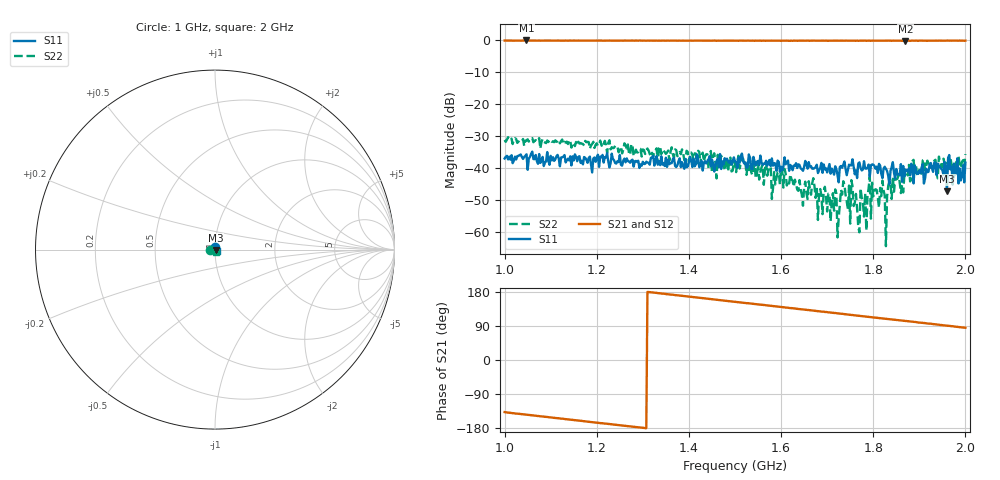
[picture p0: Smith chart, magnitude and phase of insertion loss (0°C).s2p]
!Agilent Technologies,E8363C,MY43030407,A.09.42.15
!Agilent E8363C: A.09.42.15
!Date: Friday, September 05, 2025 17:05:36
!Correction: S11(Full 2 Port(1,2))
!S21(Full 2 Port(1,2))
!S12(Full 2 Port(1,2))
!S22(Full 2 Port(1,2))
!S2P File: Measurements: S11, S21, S12, S22:
# Hz S  dB  R 50
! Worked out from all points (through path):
!   401 points, 1 GHz to 2 GHz, reference 50 ohm
!   highest |S21| = -0.06 dB at 1.048 GHz (marker M1); lowest = -0.2 dB at 1.87 GHz (marker M2)
!   group delay of S21, straight-line fit = 381 ps
!   lowest |S11| = -47.3 dB at 1.96 GHz (marker M3), VSWR 1.01, Z = 50.3 - j0.265 ohm
!   |S11| at or under -10 dB: start of sweep to end of sweep
!   |S22| runs from -64.5 to -30.3 dB; largest |S21 - S12| = 0.011
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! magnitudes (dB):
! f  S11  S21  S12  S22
! 1 GHz  -37.1  -0.1  -0.1  -31.3
! 1.048 GHz  -35.7  -0.1  -0.1  -31.4
! 1.167 GHz  -37.8  -0.1  -0.1  -32.4
! 1.335 GHz  -37.9  -0.1  -0.1  -33.8
! 1.5 GHz  -38.0  -0.1  -0.1  -39.1
! 1.653 GHz  -37.8  -0.1  -0.1  -44.3
! 1.667 GHz  -40.2  -0.1  -0.1  -44.8
! 1.685 GHz  -40.0  -0.1  -0.1  -46.6
! 1.715 GHz  -42.1  -0.1  -0.2  -53.4
! 1.72 GHz  -40.4  -0.1  -0.1  -48.0
! 1.728 GHz  -39.7  -0.1  -0.2  -51.6
! 1.735 GHz  -39.0  -0.1  -0.1  -44.2
! 1.745 GHz  -40.6  -0.1  -0.1  -52.9
! 1.758 GHz  -39.8  -0.1  -0.1  -52.0
! 1.765 GHz  -43.2  -0.1  -0.2  -52.7
! 1.792 GHz  -42.7  -0.1  -0.1  -42.7
! 1.82 GHz  -43.2  -0.1  -0.2  -44.0
! 1.827 GHz  -40.3  -0.1  -0.1  -64.5
! 1.835 GHz  -45.2  -0.1  -0.2  -44.2
! 1.87 GHz  -40.6  -0.2  -0.1  -42.2
! 1.96 GHz  -47.3  -0.1  -0.1  -38.4
! 2 GHz  -38.4  -0.1  -0.1  -35.7
